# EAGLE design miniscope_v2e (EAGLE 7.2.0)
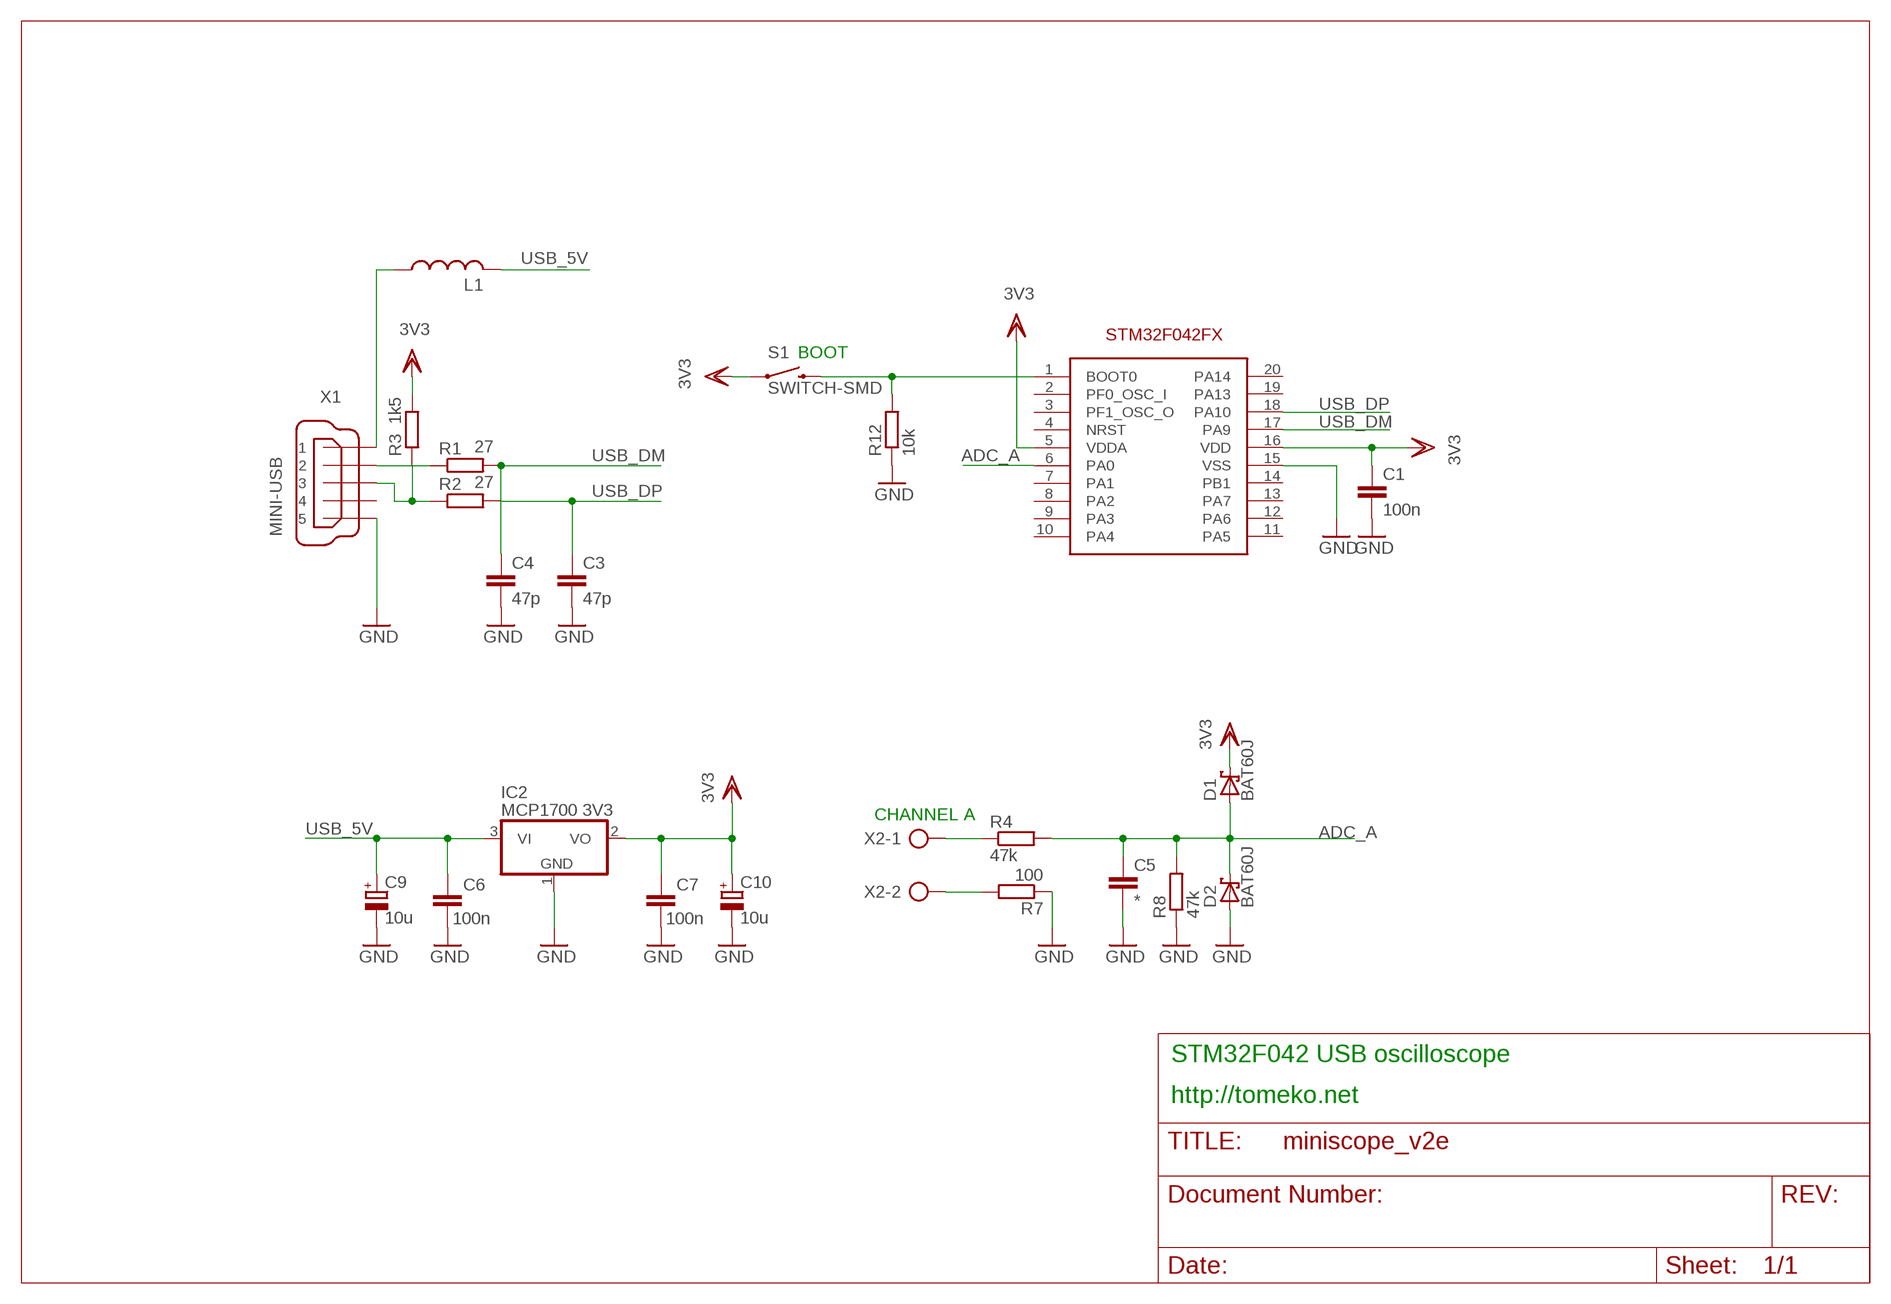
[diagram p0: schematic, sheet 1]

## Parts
C1  100n  C-EUC0805K  [C0805K]
C3  47p  C-EUC0805K  [C0805K]
C4  47p  C-EUC0805K  [C0805K]
C5  *  C-EUC0805K  [C0805K]
C6  100n  C-EUC0805K  [C0805K]
C7  100n  C-EUC0805K  [C0805K]
C9  10u  CPOL-EUCT3216  [CT3216]
C10  10u  CPOL-EUCT3216  [CT3216]
D1  BAT60J  [SOD323_ST]
D2  BAT60J  [SOD323_ST]
IC2  MCP1700 3V3  MCP1703CB  [SOT23]
L1  L-USL3216C  [L3216C]
R1  27  R-EU_R0805  [R0805_40M_SPACE]
R2  27  R-EU_R0805  [R0805_40M_SPACE]
R3  1k5  R-EU_R0805  [R0805_40M_SPACE]
R4  47k  R-EU_R0805  [R0805]
R7  100  R-EU_R0805  [R0805]
R8  47k  R-EU_R0805  [R0805]
R12  10k  R-EU_R0805  [R0805]
S1  SWITCH-SMD  SWITCH-MOMENTARY-2SMD-1101NE  [TACTILE-SWITCH-1101NE]
U1  STM32F042FX  [TSSOP20]
X1  MINI-USB  MINI-USB-32005-201  [32005-201]
X2  AK500/2  [AK500/2]

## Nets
ADC_A: C5.1 D1.A D2.C R4.2 R8.2 U1.6(PA0)
GND: C1.2 C3.2 C4.2 C5.2 C6.1 C7.1 C9.- C10.- D2.A IC2.1(GND) R7.1 R8.1 R12.1 U1.15(VSS) X1.5
N$2: R1.1 X1.2
N$4: L1.1 X1.1
N$5: R2.1 R3.1 X1.3
N$9: R12.2 S1.2 U1.1(BOOT0)
N$11: R7.2 X2.2
N$13: R4.1 X2.1
USB_5V: C6.2 C9.+ IC2.3(VI) L1.2
USB_DM: C4.1 R1.2 U1.17(PA9)
USB_DP: C3.1 R2.2 U1.18(PA10)
VDD: C1.1 C7.2 C10.+ D1.C IC2.2(VO) R3.2 S1.1 U1.5(VDDA) U1.16(VDD) ; supply symbol labelled 3V3
Unconnected: U1.2(PF0_OSC_I) U1.3(PF1_OSC_O) U1.4(NRST) U1.7(PA1) U1.8(PA2) U1.9(PA3) U1.10(PA4) U1.11(PA5) U1.12(PA6) U1.13(PA7) U1.14(PB1) U1.19(PA13) U1.20(PA14) X1.4

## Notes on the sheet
- BOOT
- CHANNEL A
- STM32F042 USB oscilloscope
- http://tomeko.net

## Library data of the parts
C1 C3-C7 = resistor:C-EU: CAPACITOR, European symbol
C9 C10 = resistor:CPOL-EU: POLARIZED CAPACITOR, European symbol
D1 D2 = diode:BAT60J: Schottky barrier diode
IC2 = linear:MCP1703: 250 mA, 16V, Low Quiescent Current LDO Regulator Source: http://ww1.microchip.com/downloads/en/DeviceDoc/22049b.pdf
L1 = resistor:L-US: INDUCTOR, American symbol
R1-R3 = resistor:R-EU_: RESISTOR, European symbol
R4 R7 R8 R12 = rcl:R-EU_: RESISTOR, European symbol
S1 = SparkFun-Electromechanical:SWITCH-MOMENTARY-2: Various NO switches- pushbuttons, reed, etc; PROD_ID: SWCH-00815
U1 = STM32F042Fx:STM32F042FX: STM32F042Fx microcontroller
X1 = con-cypressindustries:MINI-USB-: MINI USB-B Conector Source: www.cypressindustries.com; OC_FARNELL: unknown; OC_NEWARK: unknown
X2 = con-ptr500:AK500/2: CONNECTOR; OC_FARNELL: unknown; OC_NEWARK: unknown

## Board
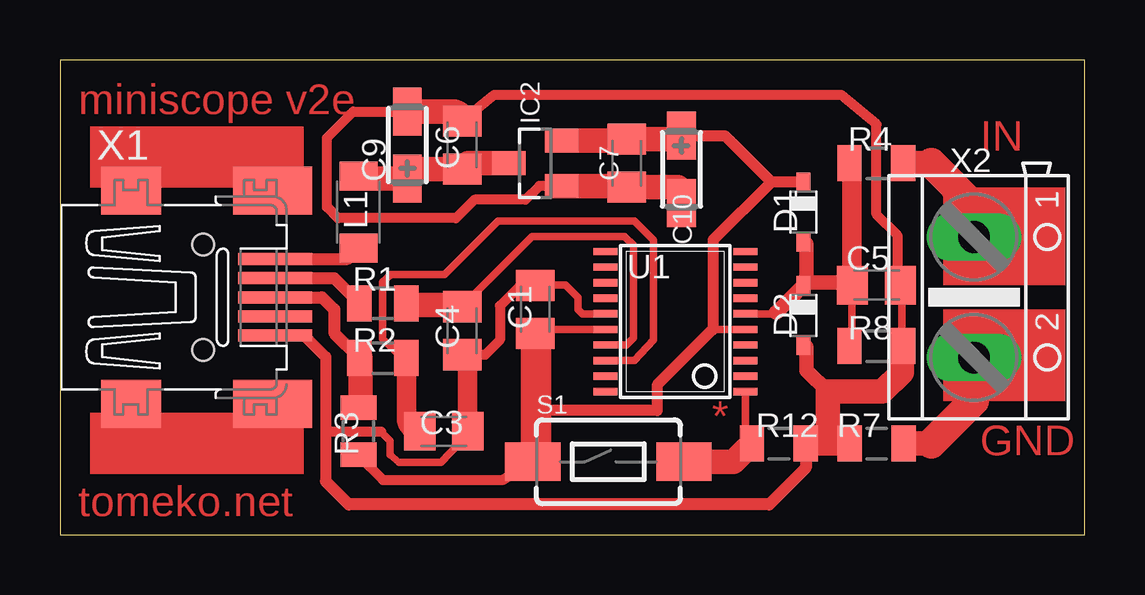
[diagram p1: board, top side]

Size 42.72 x 19.8 mm. Coordinates in mm from the lower left corner, seen from the top.
Outline: 0,0 42.72,0 42.72,19.8 0,19.8 0,0
Copper layers (1*16): Top 0.035mm / dielectric 1.5mm / Bottom 0.035mm
Design rules "default *": minimum track width 12mil, minimum drill 24mil, track to track 10mil, track to pad 9mil, pad to pad 10mil, via to via 10mil, smd to smd 10mil, copper to edge 40mil, drill to drill 8mil, minimum pad ring 10mil, minimum via ring 8mil, stop-mask expansion 4mil, vias tented up to drill 0mil, thermal gap 10mil

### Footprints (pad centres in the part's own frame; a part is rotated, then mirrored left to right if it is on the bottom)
C0805K = smd 1.3 x 1.6: 1 -1,0; 2 1,0
CT3216 = smd 2 x 1.2: + 1.4,0; - -1.4,0
SOD323_ST = smd 0.8 x 0.6: A 1.25,0; C -1.25,0
SOT23 = smd 1 x 1.4: 1 -0.95,-1.1; 2 0.95,-1.1; 3 0,1.1
L3216C = smd 1.2 x 1.6: 1 -1.5,0; 2 1.5,0
R0805_40M_SPACE = smd 1.016 x 1.5: 1 -0.977,0; 2 0.977,0
R0805 = smd 1.016 x 1.5: 1 -1.118,0; 2 1.128,0
TACTILE-SWITCH-1101NE = smd 2.3 x 1.6: 1 -3.15,0; 2 3.15,0
TSSOP20 = smd 0.305 x 0.991: 1 -2.925,-2.918; 2 -2.275,-2.918; 3 -1.625,-2.918; 4 -0.975,-2.918; 5 -0.325,-2.918; 6 0.325,-2.918; 7 0.975,-2.918; 8 1.625,-2.918; 9 2.275,-2.918; 10 2.925,-2.918; 11 2.925,2.918; 12 2.275,2.918; 13 1.625,2.918; 14 0.975,2.918; 15 0.325,2.918; 16 -0.325,2.918; 17 -0.975,2.918; 18 -1.625,2.918; 19 -2.275,2.918; 20 -2.925,2.918
32005-201 = smd 3.1 x 0.5: 1 3,1.6; 2 3,0.8; 3 3,0; 4 3,-0.8; 5 3,-1.6 | smd 2.5 x 2: M1 -3,-4.45; M2 -3,4.45 | smd 3.3 x 2: M3 2.9,4.45; M4 2.9,-4.45 | hole 0.9: 0,2.2; 0,-2.2
AK500/2 = drill 1.321 long: 1 -2.515,0; 2 2.515,0

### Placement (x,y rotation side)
C1  19.81,9.4 90 top
C3  16,4.32 0 top
C4  16.76,8.51 270 top
C5  34.04,10.41 0 top
C6  16.76,16.26 270 top
C7  23.62,15.49 90 top
C9  14.48,16.26 270 top
C10  25.91,15.24 90 top
D1  30.99,13.46 270 top
D2  30.99,9.14 270 top
IC2  19.81,15.49 90 top
L1  12.45,13.46 90 top
R1  13.46,9.65 0 top
R2  13.46,7.37 0 top
R3  12.45,4.32 270 top
R4  34.04,15.49 180 top
R7  34.04,3.81 0 top
R8  34.04,7.87 180 top
R12  29.97,3.81 180 top
S1  22.86,3.05 0 top
U1  25.65,8.89 90 top
X1  5.97,9.91 0 top
X2  38.1,9.91 270 top

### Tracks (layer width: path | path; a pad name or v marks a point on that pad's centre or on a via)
ADC_A
  Top 0.305: 31.11,10.54 D2.C 31.11,10.38 | 31.11,12.13 D1.A | R8.2 33.02,8 33.02,10.38 C5.1 | 33.02,15.46 R4.2 | 33.02,10.54 C5.1 | 32.86,10.38 C5.1 | U1.6 29.79,9.21 29.84,9.27
  Top 0.61: 29.84,9.27 29.86,9.27 D2.C 31.11,10.52 | 31.11,12.13 31.11,10.52 | 31.11,10.52 32.93,10.52 C5.1
  Top 0.813: 33.02,15.46 33.02,10.43 C5.1
GND
  Top 0.305: 16.99,7.21 16.83,7.37 C4.2 16.83,7.53 | 16.99,4.35 C3.2 16.99,4.19 15.88,3.03 14.13,3.03 13.77,3.34 13.77,3.92 13.39,4.3 | 19.68,10.38 C1.2 19.83,10.41 21.08,10.41 21.59,9.91 21.59,9.4 21.77,9.21 U1.15 | 31.11,7.84 D2.A | 35.08,7.84 R8.1 35.08,8 35.08,10.38 C5.2 34.92,10.54 | 14.53,17.73 C9.- 14.53,17.63
  Top 0.406: 19.68,10.38 19.17,10.38 18.34,9.55 18.34,8.13 17.72,7.51 C4.2 | IC2.1 19.98,14.54 19.41,13.97 17.27,13.97 16.51,13.21 11.58,13.21 11.12,13.66 11.12,16.56 12.22,17.66 C9.- | 34.92,10.54 34.92,12.47 34.04,13.36 34.04,17.12 32.56,18.34 18.1,18.34 C6.1 | 13.39,4.3 11.16,4.3 11.07,4.22
  Top 0.457: X1.5 10.19,8.31 11.07,7.42 11.07,4.22 11.07,2.23
  Top 0.508: R12.1 31.09,2.79 29.57,1.27 12.04,1.27 11.07,2.23
  Top 0.61: 31.11,7.84 31.11,6.86 32,5.97
  Top 0.813: 16.99,4.35 16.99,7.29 C4.2
  Top 1.016: R7.1 32,3.81 | 32,3.81 R12.1 | 35.08,7.84 35.08,6.76 34.29,5.97 32,5.97 32,3.81 | C10.- 25.76,14.49 C7.1 23.57,14.54 IC2.1 | C6.1 arc90 16.36,17.66 C9.-
N$2
  Top 0.508: X1.2 11.43,10.71 R1.1
N$4
  Top 0.508: X1.1 11.99,11.51 L1.1
N$5
  Top 0.305: 12.54,5.3 R3.1 | 12.54,7.37 R2.1
  Top 0.508: X1.3 10.92,9.91 11.43,9.4 11.43,8.42 R2.1
  Top 1.016: 12.54,7.37 12.54,5.39 R3.1
N$9
  Top 0.305: U1.1 28.57,4.08 R12.2
  Top 0.406: 28.59,3.56 R12.2
  Top 1.016: 28.59,3.56 28.08,3.05 S1.2
N$11
  Top 1.016: 36.32,3.81 R7.2
  Top 1.27: X2.2 38.1,5.59 36.32,3.81
N$13
  Top 1.016: 36.32,15.49 R4.1
  Top 1.27: X2.1 38.1,13.72 36.32,15.49
USB_5V
  Top 1.016: L1.2 12.55,14.86 C9.+ 14.88,15.26 C6.2 17,15.49 IC2.3
USB_DM
  Top 0.305: 14.45,9.59 R1.2 | 16.67,9.59 C4.1 16.83,9.59 19.68,12.45 23.54,12.45 23.91,12.08 23.91,8.21 23.61,7.92 U1.17
  Top 1.016: 14.45,9.59 16.68,9.59 C4.1
USB_DP
  Top 0.305: R2.2 14.29,7.37 13.44,8.16 13.44,10.54 13.81,10.86 16.03,10.86 18.26,13.08 23.95,13.08 24.75,12.29 24.74,12.28 24.74,8.13 23.94,7.26 U1.18
  Top 0.813: C3.1 arc-90 14.44,4.88 R2.2
VDD
  Top 0.305: 19.84,8.32 C1.1 19.98,8.56 U1.16 | U1.5 27.21,8.56 27.18,8.53
  Top 0.406: R3.2 12.45,3.3 13.46,2.29 18.44,2.29 S1.1
  Top 0.457: 27.18,8.53 24.89,6.25 24.89,5.18 19.84,5.18 | D1.C 29.65,14.71 | 29.65,14.71 27.23,12.29 27.23,8.59 27.21,8.56 | C10.+ 27.72,16.64 29.65,14.71
  Top 1.016: C10.+ 25.76,16.49 C7.2 23.57,16.44 IC2.2
  Top 1.27: 19.84,8.32 19.84,5.18 19.84,3.05 S1.1
(copper drawn outside any net)
  shapes: Top area x4

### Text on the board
Top: miniscope v2e | IN | * | GND | tomeko.net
